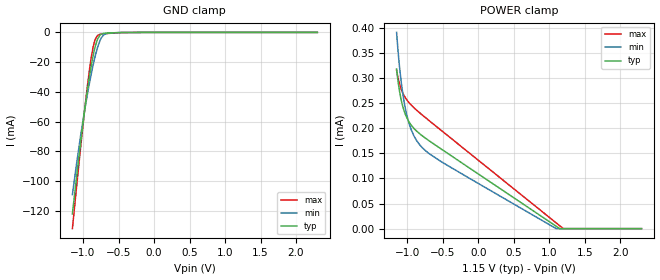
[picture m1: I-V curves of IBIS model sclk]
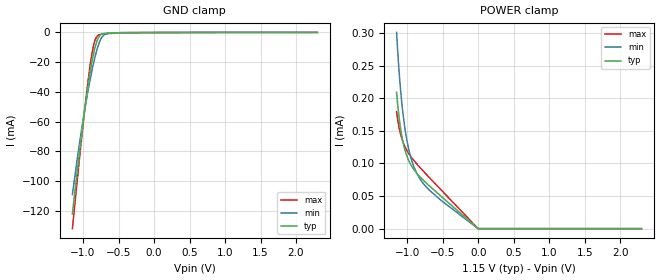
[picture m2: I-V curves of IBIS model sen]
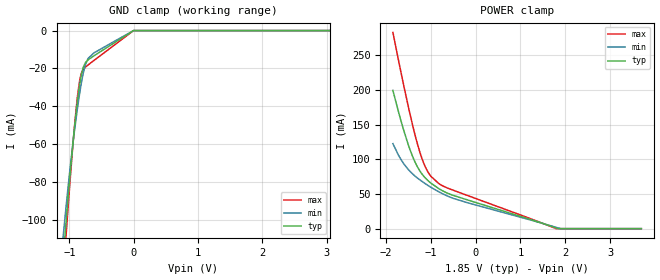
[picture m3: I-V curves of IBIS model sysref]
|Texas Instruments Incorporated
| NA
| Marketing part#   Digital Voltage Range   Package-type   #pins
| ADS54J64   1.1V-1.9V   VQFN   72
[IBIS Ver]   4.1
[File name]   ADS54J64.ibs
[File Rev]   1.0
[Date]   11/10/2016
[Source]
| Texas Instruments Incorporated.
| Analog-eLab Design Center, HPA
| 12500 TI Blvd
| Dallas, TX -75243
[Notes]   Revision History:
| Rev 1.0: 11/10/2016
| - Initial version of the model
| - Model generated from simulations in SPECTRE
| - Model matched to SPICE simulation
| - C_comp although listed in numerical order of value are
|   obtained from varying PVT conditions. For PVT conditions for
|   each specific value refer the buffer description under
|   respective [Model]. IBIS model user is responsible for using
|   appropriate C_comp to simulate for Signal Integrity.
|*EXCEPTION:   *
|* -For model sdout, sdata pullup and pulldown IV tables does not pass   *
|*  through 0 because of because of driver switch arrangement   *
|* -For model sen,there will be leakage in power and ground clamp   *
|*  IV tables because of resistors connected to pad.   *
|* -For model sclk,there will be leakage in power IV tables because   *
|*  of resistors connected to pad.   *
|* -For model sysref,there will be leakage in power IV tables because   *
|*  of transistors connected to pad.   *
|* -For model clk_in,there will be leakage in power and ground clamp   *
|*  IV tables because of transistors connected to pad.   *
[Disclaimer]
| This model is designed as an aid for customers of Texas Instruments.
| TI and its licensors and suppliers make no warranties, either expressed
| or implied, with respect to this  model, including the warranties of
| merchantability or fitness for a particular purpose. The model is
| provided solely on an "as is" basis. The entire risk as to its quality
| and performance is with the customer.
[Copyright]
(C) Copyright 2016 Texas Instruments Incorporated.All rights reserved.
|   ADS54J64RGC
[Component]   ADS54J64RGC
[Manufacturer]   TI
[Package]   |72 VQFN  -  RGC package
|   typ   min   max
R_pkg   0.10228   0.04906   0.13928
L_pkg   1.46069nH   0.69411nH   2.03974nH
C_pkg   0.22254pF   0.18927pF   0.30913pF
[Pin]  signal_name   model_name   R_pin   L_pin   C_pin
1   TRDYCD   nc   0.00160   0.07525nH  2.58435pF
2   TRIGCD   sclk   0.14263   2.08310nH  0.24742pF
3   DGND   gnd   0.12877   1.86163nH  0.22937pF
4   DVDD   power   0.05858   1.23997nH  0.26138pF
5   SDIN   sdata   0.12028   1.72653nH  0.21076pF
6   SCLK   sclk   0.13009   1.88282nH  0.22349pF
7   SEN   sen   0.11377   1.62360nH  0.19849pF
8   DVDD   power   0.11120   1.58379nH  0.20950pF
9   AVDD   power   0.11180   1.59409nH  0.20891pF
10   AVDD19   power   0.05243   0.74782nH  0.30996pF
11   SDOUT   sdout   0.10754   1.52103nH  0.20291pF
12   AVDD   power   0.06214   1.36578nH  0.28905pF
13   INDP   nc   0.14771   2.17241nH  0.25462pF
14   INDM   nc   0.13297   1.93513nH  0.23347pF
15   AVDD   power   0.14771   2.17241nH  0.25462pF
16   AVDD19   power   0.05243   0.74782nH  0.30996pF
17   AVDD   power   0.06398   1.49235nH  0.25401pF
18   INCM   nc   0.11523   1.65249nH  0.21279pF
19   INCP   nc   0.10457   1.48293nH  0.19687pF
20   AVDD   power   0.09851   1.38710nH  0.19078pF
21   AGND   gnd   0.04975   0.84853nH  0.27098pF
22   NC   nc   0.05344   1.05305nH  0.25947pF
23   NC   nc   0.10949   1.56099nH  0.20646pF
24   AVDD19   power   0.05243   0.74782nH  0.30996pF
25   AVDD   power   0.05684   1.17203nH  0.26359pF
26   AGND   gnd   0.05376   1.08583nH  0.26377pF
27   CLKINP   clk_in   0.10457   1.48293nH  0.19687pF
28   CLKINM   clk_in   0.09851   1.38710nH  0.19078pF
29   AGND   gnd   0.10052   1.41870nH  0.19282pF
30   AVDD   power   0.10918   1.55603nH  0.20559pF
31   AVDD19   power   0.05243   0.74782nH  0.30996pF
32   AGND   gnd   0.06450   1.50444nH  0.26208pF
33   SYSREFP   sysref   0.10949   1.56099nH  0.20646pF
34   SYSREFM   sysref   0.10094   1.42539nH  0.19121pF
35   AVDD   power   0.06198   1.31865nH  0.26204pF
36   INBP   nc   0.13297   1.93513nH  0.23347pF
37   INBM   nc   0.14771   2.17241nH  0.25462pF
38   AVDD   power   0.12437   1.79679nH  0.22095pF
39   AVDD19   power   0.05243   0.74782nH  0.30996pF
40   AVDD   power   0.05658   1.06733nH  0.29254pF
41   INAM   nc   0.11142   1.58779nH  0.20433pF
42   INAP   nc   0.11242   1.60249nH  0.20525pF
43   AVDD   power   0.05858   1.23997nH  0.26138pF
44   AVDD   power   0.05878   1.24561nH  0.25533pF
45   AVDD19   power   0.05243   0.74782nH  0.30996pF
46   AVDD   power   0.12028   1.72653nH  0.21076pF
47   DVDD   power   0.05858   1.23997nH  0.26138pF
48   RESET   sclk   0.13693   1.99496nH  0.22355pF
49   NC   nc   0.06330   1.47774nH  0.25634pF
50   PDN   sdata   0.12028   1.72490nH  0.22558pF
51   DVDD   power   0.05858   1.23997nH  0.26138pF
52   DGND   gnd   0.09974   1.39670nH  0.18981pF
53   TRIGAB   sclk   0.04906   0.69411nH  0.29385pF
54   TRDYAB   nc   0.04994   0.70830nH  0.30913pF
55   SYNCbABP   nc   0.10052   1.41870nH  0.19282pF
56   SYNCbABM   nc   0.10918   1.55603nH  0.20559pF
57   DVDD   power   0.05858   1.23997nH  0.26138pF
58   DAP   nc   0.12437   1.79679nH  0.22095pF
59   DAM   nc   0.11574   1.65789nH  0.20980pF
60   DGND   gnd   0.04975   0.84712nH  0.27049pF
61   DBP   nc   0.12437   1.79679nH  0.22095pF
62   DBM   nc   0.11574   1.65789nH  0.20980pF
63   DGND   gnd   0.05243   0.74782nH  0.30996pF
64   DVDD   power   0.05858   1.23997nH  0.26138pF
65   DCM   nc   0.12437   1.79679nH  0.22095pF
66   DCP   nc   0.11574   1.65789nH  0.20980pF
67   DGND   gnd   0.06399   1.47401nH  0.25253pF
68   DDM   nc   0.12437   1.79679nH  0.22095pF
69   DDP   nc   0.11574   1.65789nH  0.20980pF
70   DVDD   power   0.05858   1.23997nH  0.26138pF
71   SYNCbCDM   nc   0.10052   1.41870nH  0.19282pF
72   SYNCbCDP   nc   0.10918   1.55603nH  0.20559pF
[Diff_pin]   inv_pin   vdiff   tdelay_typ   tdelay_min   tdelay_max
27   28   200mV   NA   NA   NA
33   34   200mV   NA   NA   NA
55   56   200mV   NA   NA   NA
71   72   200mV   NA   NA   NA
| Models and submodels in the file (6): sclk (Input), sen (Input), sysref (Input), clk_in (Input), sdout (Output), sdata (I/O)
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|   sclk Model
[Model]   sclk
Model_type   Input
Vinl = 0.345
Vinh = 0.805
|   typ   min   max
|   (nom PVT)   (fast PVT)   (slow PVT)
C_comp   2.536e-17   2.536e-17   2.536e-17
| Where nom  PVT is Nominal Process, 1.15V, 27C
|   Fast PVT is Strong Process,  1.2V, -40C
|   Slow PVT is Weak Process,   1.1V, 125C
[Voltage Range]   1.15   1.1   1.2
|Junction Temperature
[Temperature Range]   27   125   -40
[Power Clamp Reference]   1.15   1.1   1.2
[GND Clamp Reference]   0   0   0
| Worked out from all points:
|   GND clamp passes 1 mA (typ) near -0.73 V on its own axis
[GND Clamp]
|   Voltage   I(typ)   I(min)   I(max)
-1.15V    -122mA     -109.1mA   -132mA
-1.027V   -71.21mA   -67.22mA   -73.97mA
-941.2mV  -39.71mA   -42.25mA   -37.11mA
-907.6mV  -29.05mA   -33.57mA   -24.55mA
-878.8mV  -20.92mA   -26.64mA   -15.36mA
-852.4mV  -14.42mA   -20.74mA   -8.734mA
-827.7mV  -9.327mA   -15.71mA   -4.557mA
-794.8mV  -4.443mA   -9.938mA   -1.989mA
-742mV    -1.195mA   -3.649mA   -1.096mA
-701.5mV  -640.1uA   -1.423mA   -894.6uA
-647.3mV  -411.8uA   -447.6uA   -685.3uA
2.3V      0A         0A         0A
[POWER Clamp]
|   Voltage   I(typ)   I(min)   I(max)
-1.15V    318.2uA    391.1uA    315.6uA
-1.118V   282uA      335.4uA    293.2uA
-1.076V   251.1uA    282.9uA    274.8uA
-1.031V   229.5uA    243uA      261.9uA
-985mV    215.2uA    214.8uA    252.7uA
-944.3mV  206.3uA    197.3uA    246.3uA
-869.4mV  194.6uA    175.9uA    236.3uA
-696.8mV  175.6uA    150uA      215.9uA
1.098V    4.791uA    40.38nA    11.43uA
1.149V    0A         0A         5.686uA
1.198V    0A         0A         45.53nA
2.3V      0A         0A         0A
|   sen Model
[Model]   sen
Model_type   Input
Vinl = 0.345
Vinh = 0.805
|   typ   min   max
|   (nom PVT)   (fast PVT)   (slow PVT)
C_comp   2.536e-17   2.536e-17   2.536e-17
| Where nom  PVT is Nominal Process, 1.15V, 27C
|   Fast PVT is Strong Process,  1.2V, -40C
|   Slow PVT is Weak Process,   1.1V, 125C
[Voltage Range]   1.15   1.1   1.2
|Junction Temperature
[Temperature Range]   27   125   -40
[Power Clamp Reference]   1.15   1.1   1.2
[GND Clamp Reference]   0   0   0
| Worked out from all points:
|   GND clamp passes 1 mA (typ) near -0.72 V on its own axis
[GND Clamp]
|   Voltage   I(typ)   I(min)   I(max)
-1.15V    -122.2mA   -109.2mA   -132.1mA
-1.027V   -71.31mA   -67.31mA   -74.11mA
-941.2mV  -39.82mA   -42.34mA   -37.25mA
-907.6mV  -29.16mA   -33.66mA   -24.69mA
-878.8mV  -21.03mA   -26.73mA   -15.49mA
-852.4mV  -14.53mA   -20.83mA   -8.871mA
-827.7mV  -9.436mA   -15.8mA    -4.693mA
-794.8mV  -4.552mA   -10.03mA   -2.125mA
-742mV    -1.305mA   -3.739mA   -1.233mA
-701.5mV  -749.3uA   -1.513mA   -1.031mA
-647.3mV  -521uA     -537.9uA   -821.9uA
2.3V      0A         0A         0A
[POWER Clamp]
|   Voltage   I(typ)   I(min)   I(max)
-1.15V    209uA      300.8uA    179uA
-1.132V   186.9uA    267.4uA    165.2uA
-1.112V   167.4uA    236.3uA    153.3uA
-1.091V   151.6uA    209.7uA    143.9uA
-1.067V   136.7uA    183.4uA    135.2uA
-1.014V   114.2uA    140.7uA    121.5uA
-948.7mV  97.91uA    108.7uA    110.3uA
-869.4mV  85.37uA    85.63uA    99.66uA
-792.4mV  76.25uA    71.75uA    90.37uA
-518.6mV  49.18uA    42.95uA    58.91uA
-500uV    0A         0A         0A
2.3V      0A         0A         0A
|   sysref Model
[Model]   sysref
Model_type   Input
Vinl = 0.555
Vinh = 1.295
|   typ   min   max
|   (nom PVT)   (fast PVT)   (slow PVT)
C_comp   2.900e-13   2.437e-13   3.469e-13
| Where nom  PVT is Nominal Process, 1.85V, 27C
|   Fast PVT is Strong Process,  1.8V, -40C
|   Slow PVT is Weak Process,   1.9V, 125C
[Voltage Range]   1.85   1.9   1.8
|Junction Temperature
[Temperature Range]   27   125   -40
[Power Clamp Reference]   1.85   1.9   1.8
[GND Clamp Reference]   0   0   0
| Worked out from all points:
|   GND clamp passes 1 mA (typ) near -0.05 V on its own axis
[GND Clamp]
|   Voltage   I(typ)   I(min)   I(max)
-1.85V    -468.5mA   -413.3mA   -514.9mA
-1.098V   -120.4mA   -109.1mA   -130.2mA
-1.067V   -107.6mA   -98.47mA   -115.7mA
-1.054V   -102.1mA   -93.98mA   -109.5mA
-1.022V   -88.62mA   -83.03mA   -94.08mA
-951.3mV  -61.68mA   -61.49mA   -62.85mA
-879.8mV  -38.73mA   -42.38mA   -36.31mA
-812.2mV  -23.25mA   -27.38mA   -22.42mA
-707mV    -15.38mA   -14.62mA   -18.1mA
-185mV    -3.95mA    -3.469mA   -4.683mA
-1.4mV    0A         -1.294uA   0A
3.7V      0A         0A         0A
[POWER Clamp]
|   Voltage   I(typ)   I(min)   I(max)
-1.85V    199.5mA    122.7mA    283.1mA
-1.663V   154.2mA    99.1mA     223.6mA
-1.506V   121mA      85.32mA    176.2mA
-1.367V   97.72mA    76.53mA    138.3mA
-1.258V   84.3mA     70.89mA    112.5mA
-1.147V   74.65mA    65.81mA    92.16mA
-1.065V   69.25mA    62.31mA    81.56mA
-824mV    57.74mA    53.18mA    65.06mA
-185mV    41.47mA    37.45mA    47.88mA
1.799V    1.067mA    1.879mA    0A
1.899V    0A         0A         0A
3.7V      0A         0A         0A
